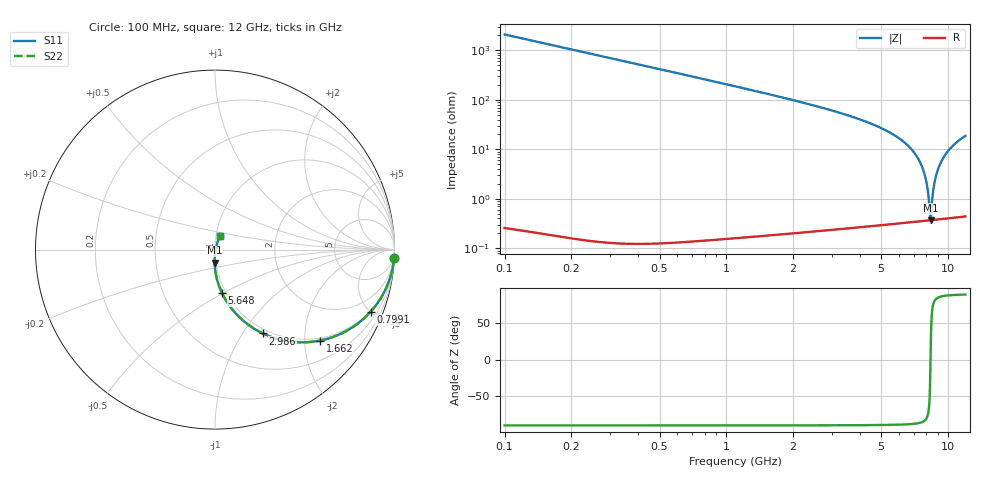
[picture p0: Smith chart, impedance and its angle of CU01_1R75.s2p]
! S-parameter model data by Modelithics Inc. support@modelithics.com 813-866-6335 Tampa FL USA
! S-Parameter data specifications:
! Substrate: 20-mil Rogers, substrate thickness, H=0.508mm, Dielectric constant, Er=3.75
! PCB Mounting Pad Footprint: Pad width, PadW=0.35mm , Pad length, PadL=0.30mm , Pad gap, PadG (edge-to-edge)=0.25mm , Reference planes=0.85mm apart
! Created Tue May  8 14:01:25 2018
# hz S ma R 50
! 2 Port Network Data from SP1.SP block
! freq  magS11  angS11  magS21  angS21  magS12  angS12  magS22  angS22
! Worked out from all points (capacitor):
!   801 points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, 100 MHz to 12 GHz, reference 50 ohm
!   read as one part in series: C = 759 fF near 159.5 MHz
!   lowest |Z| = 370 mohm at 8.356 GHz (marker M1)
!   series resonance near 8.352 GHz, so ESL is about 480 pH
!   S11 on the Smith chart (normalised r, x): 100 MHz: 1, -40; 799.1 MHz: 0.93, -5.03; 1.662 GHz: 0.93, -2.37; 2.986 GHz: 0.94, -1.24; 5.648 GHz: 0.96, -0.49; 12 GHz: 1.04, +0.16
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1e8  0.9989 -2.8  0.04762 87.2  0.04762 87.2  0.9989 -2.8
2.33875e8  0.9938 -6.6  0.1109 83.4  0.1109 83.4  0.9938 -6.6
3.6775e8  0.9849 -10.3  0.1729 79.7  0.1729 79.7  0.9849 -10.3
7.99125e8  0.9335 -21.8  0.3579 68.2  0.3579 68.2  0.9335 -21.8
1.661875e9  0.7747 -40.8  0.6311 49.1  0.6311 49.1  0.7747 -40.8
2.09325e9  0.6912 -48.3  0.7212 41.6  0.7212 41.6  0.6912 -48.3
2.98575e9  0.5382 -60.3  0.8408 29.5  0.8408 29.5  0.5382 -60.3
4.071625e9  0.394 -70.6  0.9166 19.1  0.9166 19.1  0.394 -70.6
5.648375e9  0.2442 -80.9  0.9667 8.4  0.9667 8.4  0.2442 -80.9
6.05e9  0.2136 -83.0  0.9738 6.2  0.9738 6.2  0.2136 -83.0
8.04325e9  0.08999 -90.8  0.9923 -3.0  0.9923 -3.0  0.08999 -90.8
8.355625e9  0.07371 -91.5  0.9935 -4.3  0.9935 -4.3  0.07371 -91.5
8.87625e9  0.04796 -91.8  0.995 -6.3  0.995 -6.3  0.04796 -91.8
9.263e9  0.02987 -90.4  0.9956 -7.7  0.9956 -7.7  0.02987 -90.4
9.605125e9  0.01467 -83.6  0.9959 -9.0  0.9959 -9.0  0.01467 -83.6
9.902625e9  0.004092 -25.8  0.9959 -10.0  0.9959 -10.0  0.004092 -25.8
9.962125e9  0.004204 9.9  0.9959 -10.2  0.9959 -10.2  0.004204 9.9
1.002162e10  0.005622 34.8  0.9959 -10.4  0.9959 -10.4  0.005622 34.8
1.02745e10  0.0152 63.4  0.9957 -11.3  0.9957 -11.3  0.0152 63.4
1.06315e10  0.0296 69.6  0.9953 -12.5  0.9953 -12.5  0.0296 69.6
1.121162e10  0.05238 71.0  0.9943 -14.4  0.9943 -14.4  0.05238 71.0
1.2e10  0.08185 70.1  0.9922 -16.9  0.9922 -16.9  0.08185 70.1
